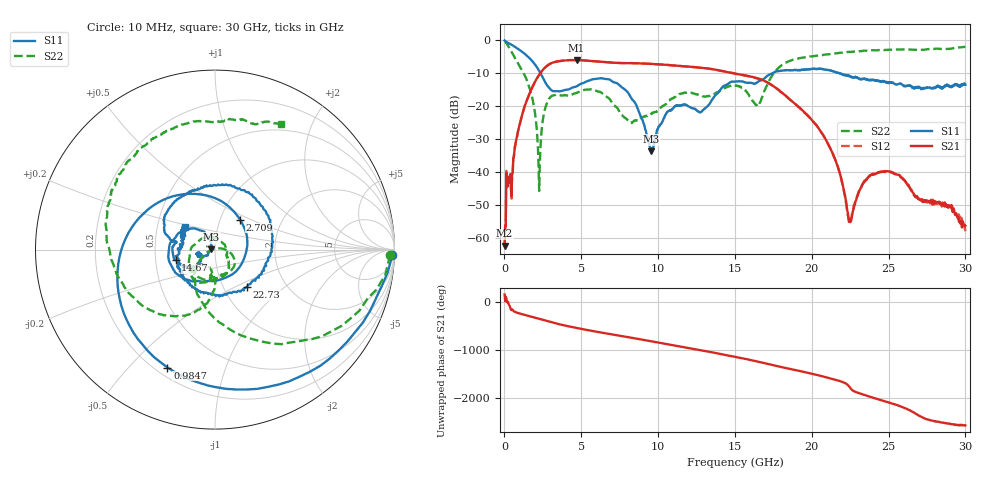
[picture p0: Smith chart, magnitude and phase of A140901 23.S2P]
!  2-Port S-parameters saved by WinCal
! VAR MeasName=S-Parameters (CALIBRATED_DATA) read from VNA (N5244A)
! VAR MeasDate=11/3/2014 9:28:43 AM
! VAR NAME=A140901 23
! VAR FILENAME=A140901 23.S2P
! VAR DATE=11/3/2014 9:28:43 AM
! VAR PHYS_PORTS=1,2
# Hz S RI R 50
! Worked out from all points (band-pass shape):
!   801 points, 10 MHz to 30 GHz, reference 50 ohm
!   highest |S21| = -6.05 dB at 4.696 GHz (marker M1); lowest = -62.3 dB at 10 MHz (marker M2)
!   |S21| within 3 dB of the highest: 2.494 GHz to 13.82 GHz (11.33 GHz wide, 139 % of centre)
!   lowest |S11| = -33.7 dB at 9.569 GHz (marker M3), VSWR 1.04, Z = 48 + j0.113 ohm
!   |S11| at or under -10 dB: 2.338 GHz to 17.46 GHz (15.13 GHz wide, 153 % of centre); 21.76967 GHz to 21.81995 GHz (50.27 MHz wide, 0.231 % of centre); 21.83 GHz to end of sweep
!   |S22| runs from -45.8 to -0.2 dB; largest |S21 - S12| = 0.0032
!   S11 on the Smith chart (normalised r, x): 10 MHz: 21, -54; 984.7 MHz: 0.25, -0.65; 2.709 GHz: 1.24, +0.44; 14.67 GHz: 0.64, -0.08; 22.73 GHz: 1.29, -0.58; 30 GHz: 0.69, +0.18
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1e7  0.9872 -0.0317  -0.000716 0.000267  0.000749 -4.96e-05  0.9752 -0.0305
4.973375e8  0.4128 -0.7343  -0.00806 -0.00494  -0.00802 -0.00474  0.3704 -0.527
9.84675e8  -0.2649 -0.6569  -0.0291 0.0428  -0.029 0.0428  0.0234 -0.4055
1.8094e9  -0.4654 0.1206  0.1202 0.1493  0.1202 0.1491  -0.0998 -0.0873
2.221762e9  -0.1689 0.3092  0.2794 0.0718  0.2789 0.072  -0.0116 0.00241
2.7091e9  0.139 0.1677  0.3424 -0.1998  0.3423 -0.199  0.0972 -0.0314
3.571312e9  0.0653 -0.154  -0.1045 -0.4697  -0.104 -0.4692  0.0673 -0.1312
4.695938e9  -0.0945 -0.1748  -0.4985 0.00102  -0.4986 0.000988  0.0135 -0.1576
5.033325e9  -0.1333 -0.1746  -0.4605 0.182  -0.4604 0.1821  -0.0175 -0.1707
6.195438e9  -0.2545 -0.0655  0.00463 0.471  0.00445 0.4709  -0.1413 -0.0828
7.582475e9  -0.1674 0.106  0.4378 0.0988  0.4375 0.0986  -0.0339 0.0668
9.569312e9  -0.0206 0.00118  -0.0646 -0.4311  -0.0647 -0.4305  0.0673 -0.0374
1.001916e10  -0.0399 -0.0265  -0.2403 -0.3568  -0.2405 -0.3563  0.0681 -0.052
1.241836e10  -0.088 -0.0188  -0.0497 0.3859  -0.0479 0.386  -0.0165 -0.152
1.466761e10  -0.2189 -0.0595  0.2396 -0.2153  0.2388 -0.2151  -0.0835 -0.1848
1.5005e10  -0.2336 -0.027  0.1401 -0.2774  0.1375 -0.2771  -0.1115 -0.1717
1.65045e10  -0.2277 0.0464  -0.2531 -0.0669  -0.2534 -0.0657  -0.0392 -0.0948
2.002832e10  0.064 0.363  0.0301 -0.0526  0.0309 -0.0521  -0.5556 -0.1106
2.242752e10  0.2445 -0.1569  0.00141 0.00103  0.00142 0.00117  -0.5743 0.3275
2.272742e10  0.1785 -0.2087  0.00137 -0.00242  0.00144 -0.00277  -0.5463 0.3816
2.501416e10  -0.1913 -0.1125  0.00516 0.00877  0.00514 0.00895  -0.272 0.6606
3e10  -0.1697 0.1257  0.000754 -0.00133  0.000452 -0.00118  0.3673 0.7012
